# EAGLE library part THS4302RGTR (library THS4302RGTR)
2.4GHz, Wideband Fixed Gain Amplifier Source: Datasheet
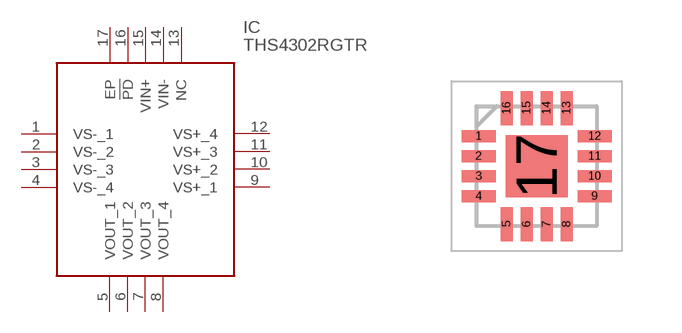
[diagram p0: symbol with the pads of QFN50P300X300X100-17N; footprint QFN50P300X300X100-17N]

Designator prefix IC

## THS4302RGTR (Description: 2.4GHz, Wideband Fixed Gain Amplifier; Height: 1mm; Manufacturer_Name: Texas Instruments; Manufacturer_Part_Number: THS4302RGTR; Mouser_Part_Number: 595-THS4302RGTR; Mouser_Price-Stock: https://www.mouser.co.uk/ProductDetail/Texas-Instruments/THS4302RGTR?qs=ZmJdcv7QZ9roaRyFJKAg2g%3D%3D)  [QFN50P300X300X100-17N]
1  VS-_1
2  VS-_2
3  VS-_3
4  VS-_4
5  VOUT_1
6  VOUT_2
7  VOUT_3
8  VOUT_4
9  VS+_1
10  VS+_2
11  VS+_3
12  VS+_4
13  NC  nc
14  VIN-
15  VIN+
16  !PD
17  EP

## Footprint QFN50P300X300X100-17N (pad centres in mm)
RGT0016A+
smd 0.85 x 0.3: 1 -1.45,0.75; 2 -1.45,0.25; 3 -1.45,-0.25; 4 -1.45,-0.75; 9 1.45,-0.75; 10 1.45,-0.25; 11 1.45,0.25; 12 1.45,0.75
smd 0.3 x 0.85: 5 -0.75,-1.45; 6 -0.25,-1.45; 7 0.25,-1.45; 8 0.75,-1.45; 13 0.75,1.45; 14 0.25,1.45; 15 -0.25,1.45; 16 -0.75,1.45
smd 1.55 x 1.55: 17 0,0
